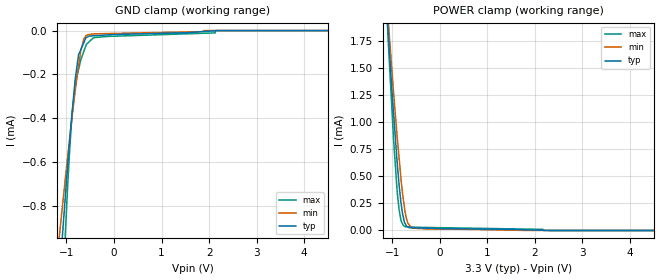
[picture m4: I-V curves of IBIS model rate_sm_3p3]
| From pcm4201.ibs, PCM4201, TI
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|   rate_sm_3p3 Model
[Model]   rate_sm_3p3
Model_type   Input
Vinl = 0.99
Vinh = 2.31
|   typ   min   max
|   (nom PVT)   (fast PVT)   (slow PVT)
|C_comp from frequency sweep method (F=27.65Hz)
|Average
|C_comp   9.427e-13   8.289e-13   1.070e-12
|C_comp from LC tank measurement(L=1nH)
|Average
|Resonant Frequency(Hz)   9.295e+10   9.541e+10   8.156e+10
C_comp   2.935e-15   2.785e-15   3.812e-15
| Where nom  PVT is Nominal Process, 3.3V, 35C
|   Fast PVT is Strong Process,  3.6V, -10C
|   Slow PVT is Weak Process,   3V, 80C
[Model Spec]
Vinl   0.99   0.9   1.08
Vinh   2.31   2.1   2.52
[Voltage Range]   3.3   3   3.6
|Ambient Temperature   25   70   -10
|Junction Temperature
[Temperature Range]   35   80   -10
[Power Clamp Reference]   3.3   3   3.6
[GND Clamp Reference]   0   0   0
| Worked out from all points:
|   GND clamp passes 1 mA (typ) near -1.11 V on its own axis
|   POWER clamp passes 1 mA (typ) near -0.96 V on its own axis
[GND Clamp]
|   Voltage   I(typ)   I(min)   I(max)
-3.3V     -7.983mA   -5.73mA    -12.93mA
-1.142V   -1.108mA   -925.5uA   -1.491mA
-1.076V   -915.7uA   -787.6uA   -1.17mA
-1.003V   -700.9uA   -636.5uA   -842.1uA
-896.4mV  -410.8uA   -422.1uA   -429.2uA
-815.1mV  -222.6uA   -273.6uA   -258uA
-745.8mV  -111.7uA   -161.2uA   -179.4uA
-696mV    -86.45uA   -90.19uA   -132.8uA
-549mV    -28.3uA    -18.48uA   -56.63uA
-414mV    -23.63uA   -14.94uA   -32.01uA
2.135V    -517nA     0A         0A
6.6V      0A         0A         0A
[POWER Clamp]
|   Voltage   I(typ)   I(min)   I(max)
-3.3V     18.4mA     16.38mA    23.06mA
-1.125V   2.099mA    2.188mA    2.126mA
-1.073V   1.745mA    1.876mA    1.66mA
-972mV    1.084mA    1.282mA    845.6uA
-896.4mV  629.3uA    868.7uA    361.7uA
-856.8mV  427.8uA    677.8uA    195.8uA
-817.2mV  261.3uA    486.9uA    97.84uA
-782.1mV  153.5uA    341.8uA    58.76uA
-738mV    73.83uA    195.1uA    37.68uA
-672mV    33.03uA    68.08uA    32.78uA
-585mV    25.01uA    21.78uA    31.39uA
6.6V      0A         0A         0A
